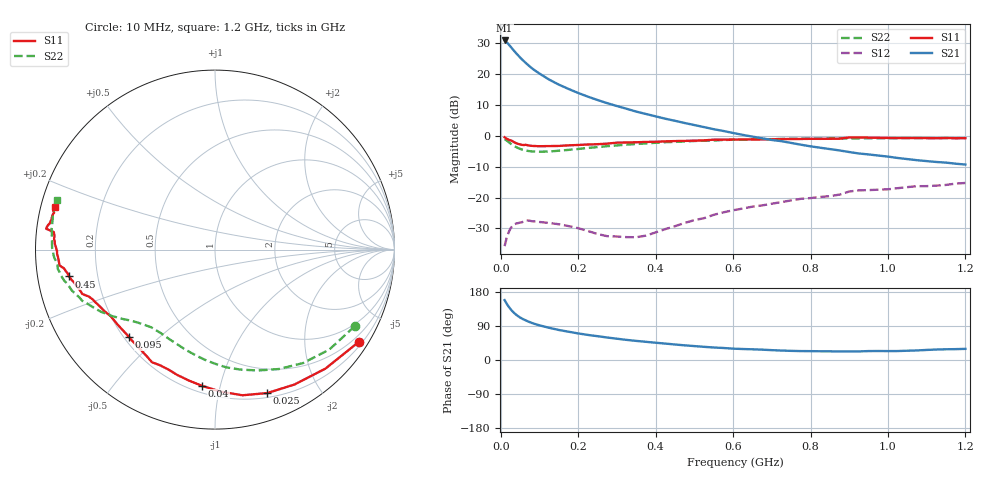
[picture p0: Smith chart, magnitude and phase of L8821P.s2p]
!  POLYFET RF DEVICES
!  L8821P S-PARAMETERS
!  Vds=12.5V,Idq=200ma,Vgs=2.7V
# MHZ  S  MA  R  50.0000
! SCATTERING PARAMETERS :
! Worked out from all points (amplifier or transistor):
!   63 points, 10 MHz to 1.2 GHz, reference 50 ohm
!   highest |S21| = 31.0 dB at 10 MHz (marker M1)
!   |S21| within 3 dB of that: start of sweep to 32 MHz
!   unconditionally stable (mu >= 1): 267.4 MHz to 452.7 MHz
!   at 60 MHz: K = 0.16, MSG = 26.0 dB, |S12| = -27.7 dB
!   at 425 MHz: K = 1.06, MAG = 16.4 dB, |S12| = -30.2 dB
!   at 1.2 GHz: K = 0.94, MSG = 3.0 dB, |S12| = -15.2 dB
!   S11 on the Smith chart (normalised r, x): 10 MHz: 0.31, -3.40; 25 MHz: 0.24, -1.40; 40 MHz: 0.24, -0.88; 95 MHz: 0.22, -0.40; 450 MHz: 0.10, -0.09; 1.2 GHz: 0.04, +0.13
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10  0.9529 -32.5  35.35 158.1  0.01634 67.6  0.8876 -28.8
15  0.9047 -47.1  33.2 149.2  0.02201 59.1  0.8459 -41.2
20  0.8725 -59.5  30.72 141.4  0.02696 51.1  0.8001 -52.2
25  0.8506 -70.0  28.23 134.6  0.03145 45.6  0.755 -61.8
30  0.8258 -79.3  25.89 128.8  0.03487 41.3  0.7152 -70.3
35  0.7916 -87.8  23.77 123.8  0.03679 36.5  0.6834 -78.0
40  0.7627 -95.3  21.88 119.3  0.03807 32.3  0.6591 -84.5
50  0.7289 -106.9  18.76 112.2  0.03942 26.9  0.6175 -95.0
60  0.7134 -115.5  16.25 106.7  0.0411 22.4  0.5896 -103.2
75  0.6975 -125.4  13.4 99.9  0.04226 17.4  0.5666 -112.3
95  0.6829 -134.5  10.79 93.0  0.04102 12.6  0.5551 -120.9
125  0.6851 -142.7  8.208 85.0  0.03885 9.2  0.5595 -129.1
150  0.6893 -147.5  6.799 79.2  0.03705 8.0  0.5764 -133.6
175  0.7043 -150.7  5.785 74.6  0.03462 7.4  0.5949 -137.1
225  0.7269 -156.0  4.338 66.2  0.02878 11.1  0.6395 -142.7
325  0.7845 -162.9  2.76 53.1  0.0229 43.2  0.7231 -151.3
425  0.8177 -168.2  1.904 43.3  0.03089 78.2  0.792 -158.8
450  0.8261 -169.6  1.762 40.9  0.03441 82.3  0.8007 -160.5
625  0.8761 -177.5  1.042 29.0  0.06657 91.9  0.8742 -171.7
825  0.8975 175.1  0.6444 23.0  0.1024 91.1  0.9085 178.1
1025  0.9255 169.5  0.4397 23.6  0.1424 89.7  0.9199 169.5
1200  0.9214 165.0  0.3439 29.4  0.173 86.9  0.9235 162.6
